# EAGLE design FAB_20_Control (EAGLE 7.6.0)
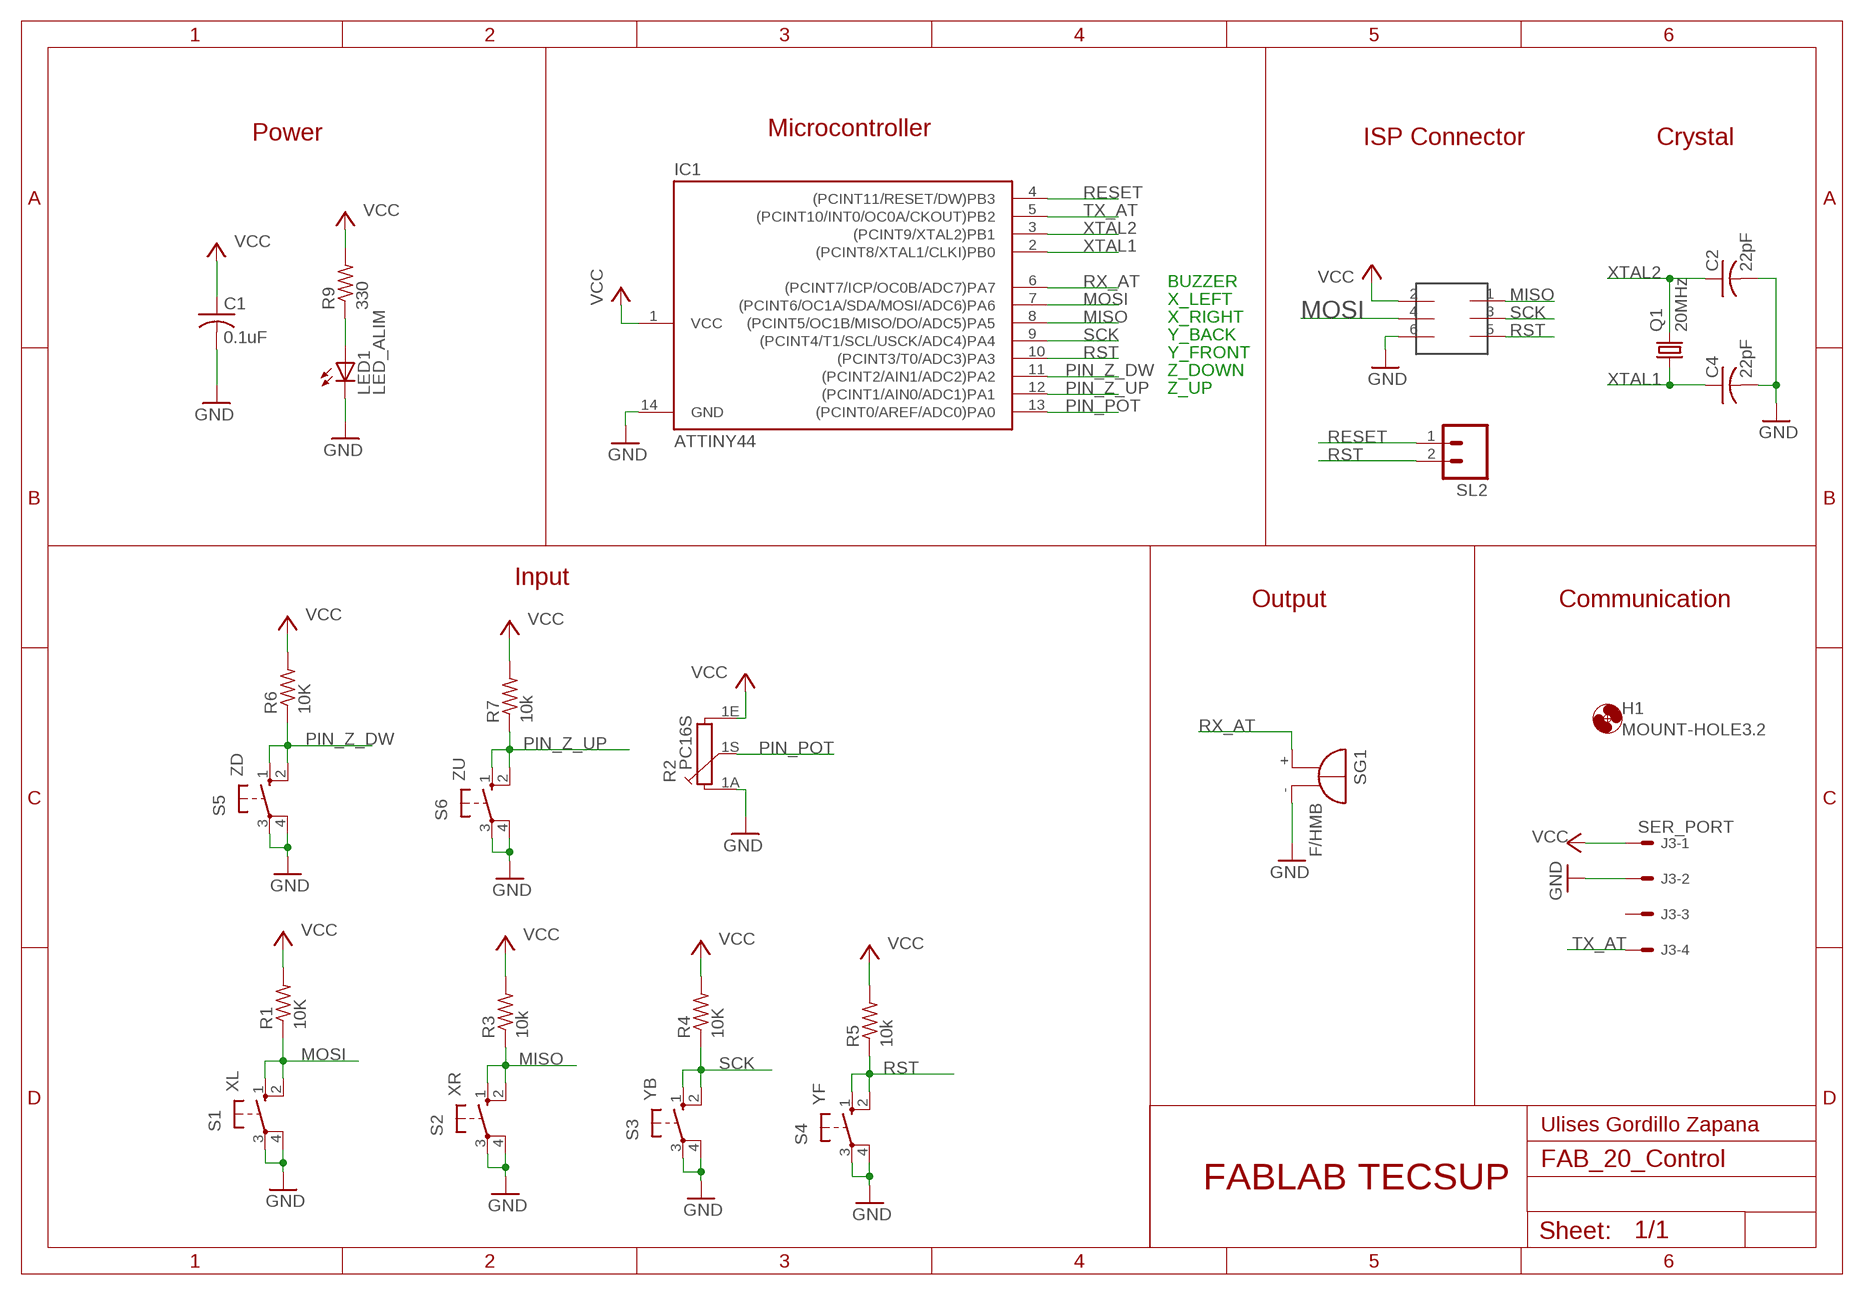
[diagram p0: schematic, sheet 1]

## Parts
C1  0.1uF  C-USC1206  [C1206]
C2  22pF  C-US025-030X050  [C025-030X050]
C4  22pF  C-US025-030X050  [C025-030X050]
H1  MOUNT-HOLE3.2  [3,2]
IC1  ATTINY44  ATTINY24/44/84-SSU  [SOIC14]
J3  SER_PORT  22-05-7048-04  [7395-04]
LED1  LED_ALIM  LED3MM  [LED3MM]
Q1  20MHz  CRYSTALHC49U-V  [HC49U-V]
R1  10K  R-US_R1206  [R1206]
R2  PC16S  [PC16S]
R3  10k  R-US_R1206  [R1206]
R4  10K  R-US_R1206  [R1206]
R5  10k  R-US_R1206  [R1206]
R6  10K  R-US_R1206  [R1206]
R7  10k  R-US_R1206  [R1206]
R9  330  R-US_R1206  [R1206]
S1  XL  10-XX  [B3F-10XX]
S2  XR  10-XX  [B3F-10XX]
S3  YB  10-XX  [B3F-10XX]
S4  YF  10-XX  [B3F-10XX]
S5  ZD  10-XX  [B3F-10XX]
S6  ZU  10-XX  [B3F-10XX]
SG1  F/HMB  [F/HMB]
SL2  M02  [02P]
U$1  2X3HEADER  [2X3_SMD]

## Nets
GND: C1.2 C2.2 C4.2 IC1.14(GND) J3.2 LED1.K(C) R2.1A S1.3(P) S1.4(P1) S2.3(P) S2.4(P1) S3.3(P) S3.4(P1) S4.3(P) S4.4(P1) S5.3(P) S5.4(P1) S6.3(P) S6.4(P1) SG1.- U$1.6
MISO: IC1.8((PCINT5/OC1B/MISO/DO/ADC5)PA5) R3.1 S2.1(S) S2.2(S1) U$1.1
MOSI: IC1.7((PCINT6/OC1A/SDA/MOSI/ADC6)PA6) R1.1 S1.1(S) S1.2(S1) U$1.4
N$8: LED1.A R9.1
PIN_POT: IC1.13((PCINT0/AREF/ADC0)PA0) R2.1S
PIN_Z_DW: IC1.11((PCINT2/AIN1/ADC2)PA2) R6.1 S5.1(S) S5.2(S1)
PIN_Z_UP: IC1.12((PCINT1/AIN0/ADC1)PA1) R7.1 S6.1(S) S6.2(S1)
RESET: IC1.4((PCINT11/RESET/DW)PB3) SL2.1
RST: IC1.10((PCINT3/T0/ADC3)PA3) R5.1 S4.1(S) S4.2(S1) SL2.2 U$1.5
RX_AT: IC1.6((PCINT7/ICP/OC0B/ADC7)PA7) SG1.+
SCK: IC1.9((PCINT4/T1/SCL/USCK/ADC4)PA4) R4.1 S3.1(S) S3.2(S1) U$1.3
TX_AT: IC1.5((PCINT10/INT0/OC0A/CKOUT)PB2) J3.4
VCC: C1.1 IC1.1(VCC) J3.1 R1.2 R2.1E R3.2 R4.2 R5.2 R6.2 R7.2 R9.2 U$1.2
XTAL1: C4.1 IC1.2((PCINT8/XTAL1/CLKI)PB0) Q1.1
XTAL2: C2.1 IC1.3((PCINT9/XTAL2)PB1) Q1.2
Unconnected: J3.3

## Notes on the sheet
- Power | Microcontroller
- ISP Connector | Crystal
- BUZZER
- X_LEFT
- X_RIGHT
- Y_BACK
- Y_FRONT
- Z_DOWN
- Z_UP
- Input
- Output | Communication
- Ulises Gordillo Zapana
- FABLAB TECSUP

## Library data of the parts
C1 = rcl-ez:C-US: CAPACITOR, American symbol
C2 C4 = rcl:C-US: CAPACITOR, American symbol
H1 = holes:MOUNT-HOLE: MOUNTING HOLE with drill center marker
IC1 = attiny24_44_84:ATTINY24/44/84
J3 = con-molex:22-?-04: CONNECTOR wire to board 2.54 mm (.1 inch) pitch header; OC_FARNELL: unknown; OC_NEWARK: unknown
LED1 = led:LED: LED
Q1 = crystal:CRYSTAL: CRYSTAL; OC_FARNELL: 1666969; OC_NEWARK: unknown
R1 R3-R7 R9 = rcl:R-US_: RESISTOR, American symbol
R2 = piher:PC16S: POTENTIOMETER single carbon potentiometer, 16 mm, S3ROH; OC_FARNELL: 4452940; OC_NEWARK: unknown
S1-S6 = switch-omron:10-XX: OMRON SWITCH; MPN: B3F-1000; OC_FARNELL: 176432; OC_NEWARK: 36M3542
SG1 = buzzer:F/HMB: BUZZER; OC_FARNELL: unknown; OC_NEWARK: unknown
SL2 = con-amp-quick:M02: AMP QUICK CONNECTOR; OC_FARNELL: unknown; OC_NEWARK: unknown
U$1 = mellis:2X3HEADER

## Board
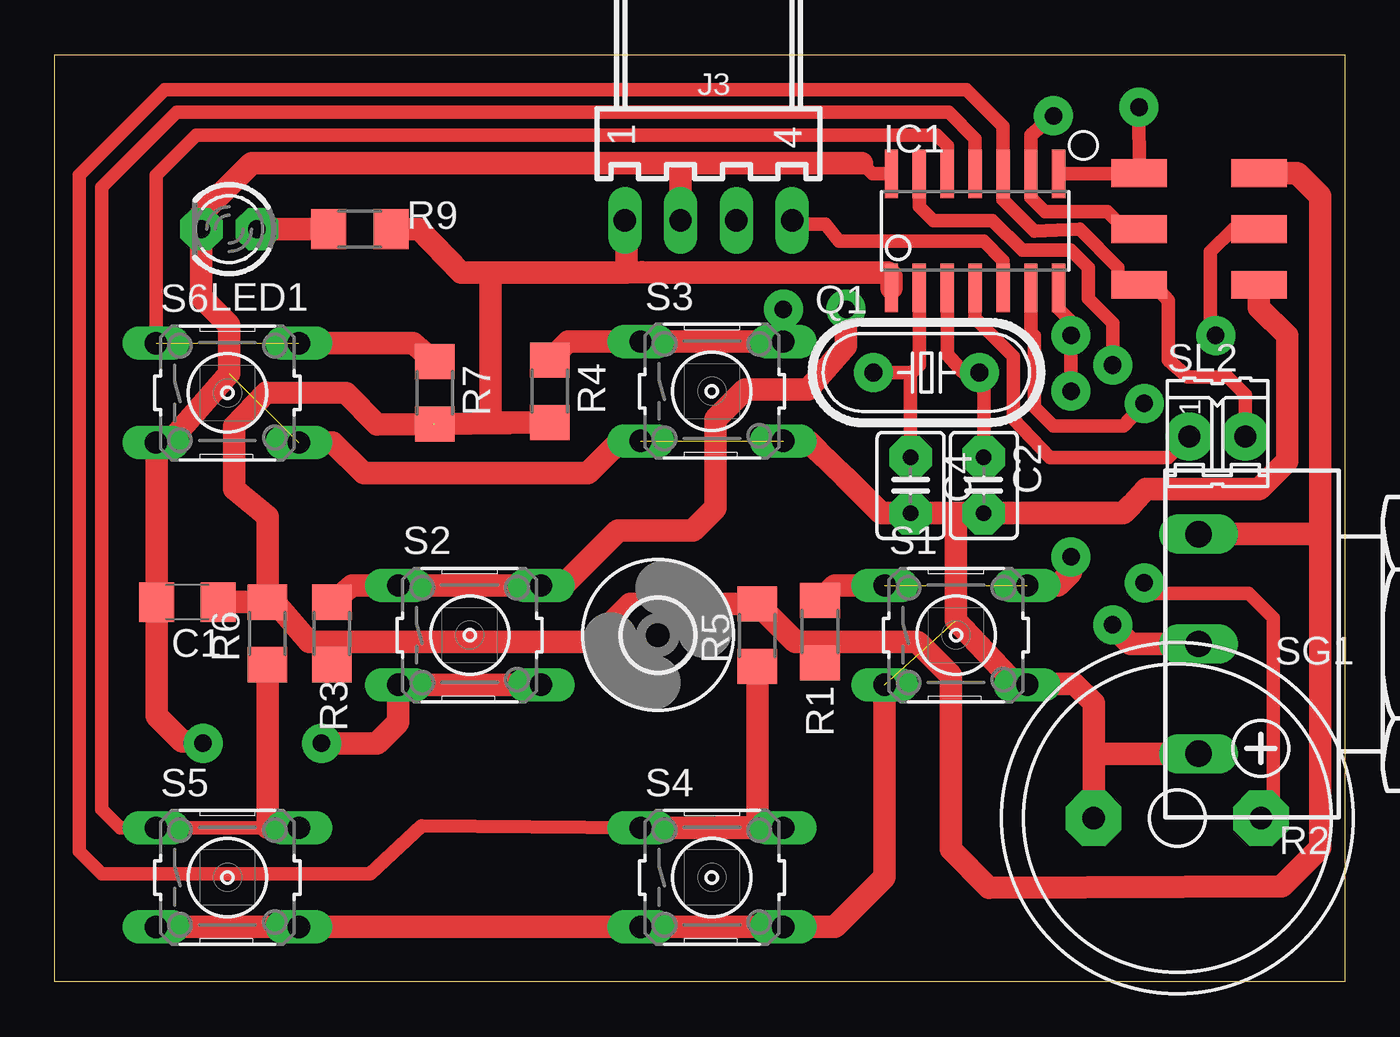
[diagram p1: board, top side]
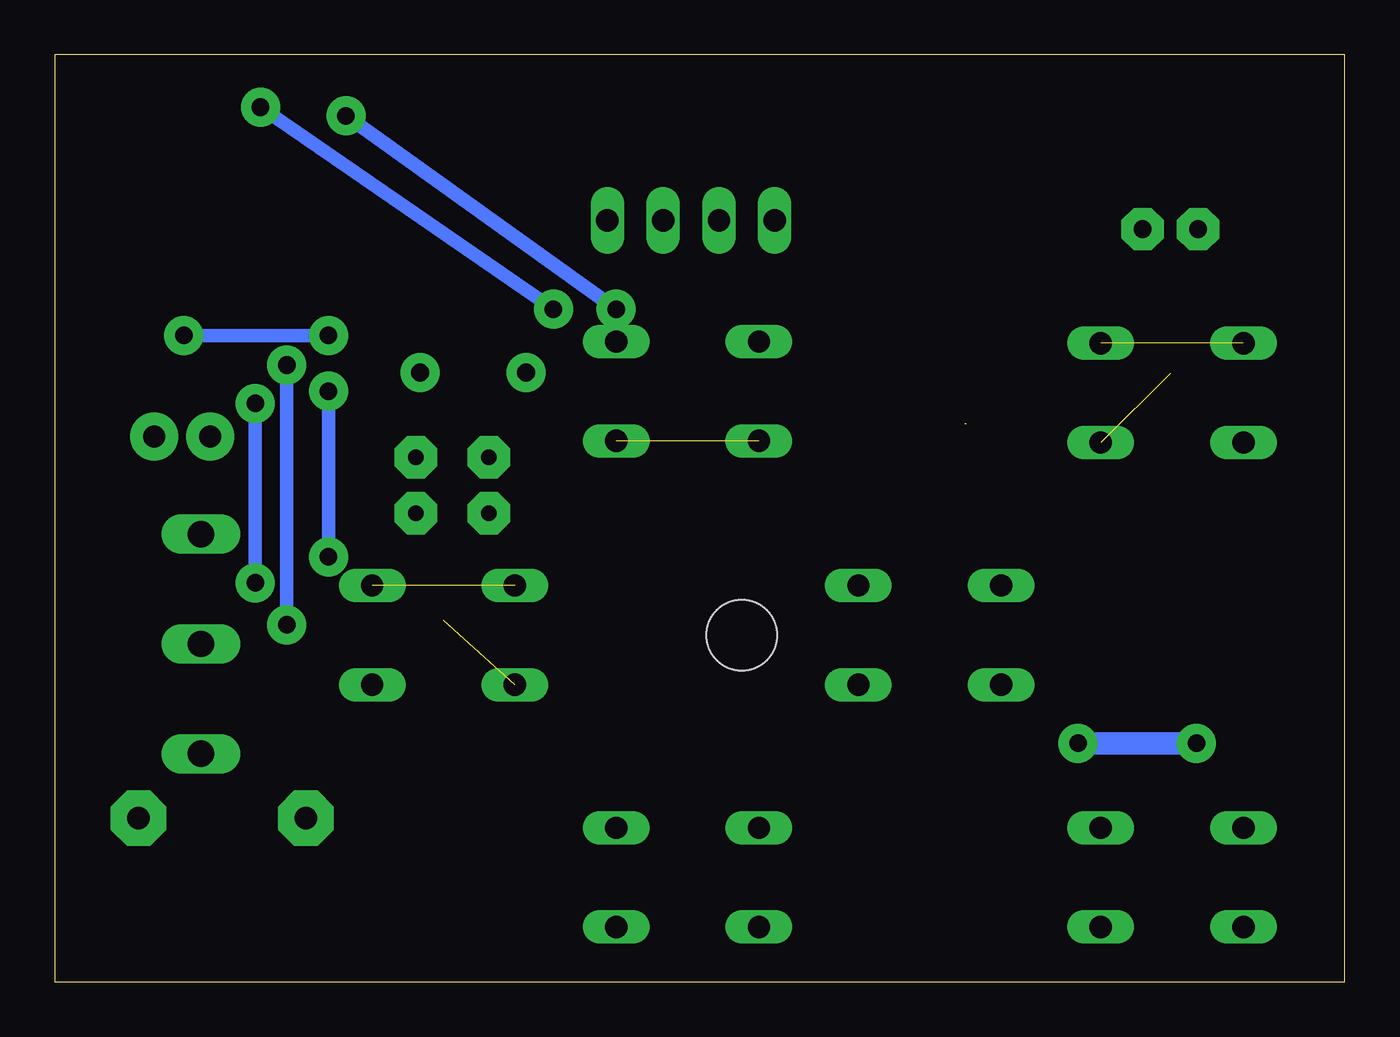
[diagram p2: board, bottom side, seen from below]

Size 58.74 x 42.23 mm. Coordinates in mm from the lower left corner, seen from the top.
Outline: 0,42.23 58.74,42.23 58.74,0 0,0 0,42.23
Copper layers (1*16): Top 0.035mm / dielectric 1.5mm / Bottom 0.035mm
Design rules "default *": minimum track width 12mil, minimum drill 24mil, track to track 17mil, track to pad 16mil, pad to pad 16mil, via to via 16mil, smd to smd 0mil, copper to edge 17mil, drill to drill 8mil, minimum pad ring 10mil, minimum via ring 8mil, stop-mask expansion 4mil, vias tented up to drill 0mil, thermal gap 10mil

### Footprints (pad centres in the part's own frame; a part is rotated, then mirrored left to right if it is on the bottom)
C1206 = smd 1.6 x 1.8: 1 -1.4,0; 2 1.4,0
C025-030X050 = drill 0.7 pad 1.93 octagon: 1 -1.27,0; 2 1.27,0
3,2 = hole 3.2: 0,0
SOIC14 = smd 0.61 x 2.21: 1 -3.81,-2.603; 2 -2.54,-2.603; 3 -1.27,-2.603; 4 0,-2.603; 5 1.27,-2.603; 6 2.54,-2.603; 7 3.81,-2.603; 8 3.81,2.603; 9 2.54,2.603; 10 1.27,2.603; 11 0,2.603; 12 -1.27,2.603; 13 -2.54,2.603; 14 -3.81,2.603
7395-04 = drill 1.016 long: 1 3.81,0; 2 1.27,0; 3 -1.27,0; 4 -3.81,0
LED3MM = drill 0.8 pad 1.93 octagon: A -1.27,0; K 1.27,0
HC49U-V = drill 0.813 pad 1.778: 1 -2.413,0; 2 2.413,0
R1206 = smd 1.6 x 1.803: 1 -1.422,0; 2 1.422,0
PC16S = drill 1.2 long: 1A -5,6.5; 1E 5,6.5; 1S 0,6.5
B3F-10XX = drill 1.016 long: 1 -3.251,2.261; 2 3.251,2.261; 3 -3.251,-2.261; 4 3.251,-2.261
F/HMB = drill 1.016 pad 2.54 octagon: + 3.81,0; - -3.81,0
02P = drill 1 pad 2.184: 1 -1.27,0; 2 1.27,0
2X3_SMD = smd 2.54 x 1.27: 1 -2.54,2.54; 2 2.92,2.54; 3 -2.54,0; 4 2.92,0; 5 -2.54,-2.54; 6 2.92,-2.54

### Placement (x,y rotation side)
C1  6.03,17.3 180 top
C2  42.31,22.62 270 top
C4  38.97,22.62 270 top
H1  27.46,15.8 0 top
IC1  41.91,34.21 0 top
J3  29.77,34.69 180 top
LED1  7.94,34.29 180 top
Q1  39.69,27.77 0 top
R1  34.85,15.95 270 top
R2  58.58,15.4 90 top
R3  12.62,15.88 270 top
R4  22.54,26.91 270 top
R5  31.99,15.8 90 top
R6  9.68,15.88 90 top
R7  17.3,26.83 270 top
R9  13.89,34.29 0 top
S1  41.04,15.8 0 top
S2  18.89,15.8 0 top
S3  29.92,26.91 0 top
S4  29.92,4.76 0 top
S5  7.86,4.76 0 top
S6  7.86,26.83 0 top
SG1  51.12,7.46 0 top
SL2  52.94,24.84 0 top
U$1  51.92,34.29 0 top

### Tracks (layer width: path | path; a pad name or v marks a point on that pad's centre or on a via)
GND  (via drill 0.8 pad 1.78)  (3 unrouted)
  Top 0.61: 44.33,13.57 S1.4 | IC1.14 37.24,36.81 36.75,37.31
  Top 1.016: R2.1A 47.31,10.4 | 47.31,10.4 47.31,12.7 46.43,13.57 44.33,13.57 | S5.3 S5.4 S4.3 S4.4 35.52,2.5 37.78,4.76 S1.3 | U$1.6 54.84,30.73 56.12,29.45 56.12,23.73 54.85,22.46 49.69,22.46 49.05,21.75 48.66,21.35 C2.2 41.04,21.35 | 28.5,37.29 8.95,37.29 6.67,35 LED1.K 6.67,31.19 7.94,29.92 7.94,27.7 5.16,24.53 4.65,24.53 S6.3 4.63,24.54 C1.2 4.63,12.12 5.79,10.95 6.67,10.95 v6.75,10.87 | J3.2 28.5,37.29 | S1.4 43.74,13.57 41.04,16.47 41.04,21.35 | v12.14,10.87 14.68,10.87 15.64,11.83 S2.3 S2.4 | S6.4 12.66,24.57 14.05,23.18 24.29,23.18 25.72,24.61 26.63,24.61 S3.3 | 36.75,37.31 28.51,37.31 28.5,37.29 | SG1.- 47.31,10.4 | 41.04,21.35 C4.2 37.62,21.35 35.96,23.02 34.77,24.17 34.29,24.65 S3.4
  Bottom 1.016: v12.14,10.87 v6.75,10.87
MISO  (via drill 0.8 pad 1.78)
  Top 0.61: IC1.8 49.04,36.81 U$1.1 v49.37,39.85
  Top 1.016: R3.1 13.54,18.06 S2.1 S2.2 23.14,18.06 25.64,20.56 29.05,20.56 30.08,21.59 30.08,25.64 31.43,26.99 34.29,26.99 36.04,28.97 v36.04,30.64
  Bottom 0.61: v36.04,30.64 v49.37,39.85
MOSI  (via drill 0.8 pad 1.78)  (1 unrouted)
  Top 0.61: U$1.4 53.66,34.29 52.63,33.26 52.63,29.69 v52.86,29.45 | v46.28,29.45 46.2,30.16 45.72,30.64 IC1.7 | v46.28,26.91 v46.28,29.45 | 46.28,29.69 v46.28,29.45
  Top 1.016: S1.1 35.52,18.06 R1.1 | S1.2 45.68,18.06 46.28,18.65 v46.28,19.37
  Bottom 0.61: v52.86,29.45 v46.28,29.45 | v46.28,19.37 v46.28,26.91
N$8
  Top 1.016: R9.1 LED1.A
PIN_POT  (via drill 0.8 pad 1.78)
  Top 0.61: IC1.13 39.37,35.32 40.01,34.69 42.7,34.69 44.05,33.34 46.28,33.34 47.07,32.54 47.07,31.11 48.18,30 v48.18,28.1
  Top 1.016: v48.18,16.27 48.18,16.19 48.97,15.4 R2.1S
  Bottom 0.61: v48.18,28.1 v48.18,16.27
PIN_Z_DW
  Top 0.61: IC1.11 41.91,38.42 40.72,39.61 5.56,39.61 2.14,36.2 2.14,7.86 2.98,7.02 S5.1 S5.2
  Top 1.016: R6.1 9.68,7.02 S5.2
PIN_Z_UP  (1 unrouted)
  Top 0.61: IC1.12 40.64,38.1 40.16,38.58 6.43,38.58 4.61,36.75 S6.1
  Top 1.016: S6.2 16.31,29.09 R7.1
RESET
  Top 0.61: IC1.4 41.91,30.24 43.66,28.5 43.66,25.64 45.32,23.89 50.72,23.89 SL2.1
RST
  Top 0.61: 49.05,31.75 48.42,31.75 48.42,32.54 46.67,34.29 44.61,34.21 43.18,35.64 IC1.10 43.18,38.97 41.51,40.64 5,40.64 1.11,36.75 1.11,5.95 2.14,4.92 14.37,4.92 16.71,7.1 S4.1 | 49.05,31.75 49.06,31.75 | 49.06,31.75 U$1.5 49.05,31.75 | SL2.2 54.21,26.75 53.42,27.54 51.59,27.54 50.72,28.34 50.72,31.04 50.01,31.83 49.21,31.83 49.13,31.75 49.06,31.75
  Top 1.016: S4.1 28.22,7.02 | 28.22,7.02 31.99,7.06 R5.1 | S4.2 28.22,7.02
RX_AT  (via drill 0.8 pad 1.78)
  Top 0.61: IC1.6 44.45,29.61 44.61,29.45 44.61,26.19 45.48,25.32 48.66,25.32 v49.61,26.35 | v49.61,18.18 50.01,17.7 54.37,17.7 55.48,16.59 55.48,8.02 SG1.+
  Bottom 0.61: v49.61,26.35 v49.61,18.18
SCK  (via drill 0.8 pad 1.78)
  Top 0.61: U$1.3 49.06,34.29 48.74,34.29 47.94,35.08 45.09,35.08 44.45,35.72 IC1.9 44.45,38.58 v45.48,39.45
  Top 1.016: v33.18,30.64 S3.2 S3.1 23.38,29.17 R4.1
  Bottom 0.61: v33.18,30.64 v45.48,39.45
TX_AT
  Top 0.61: IC1.5 43.18,32.86 42.31,33.73 35.72,33.73 35.08,34.53 33.73,34.53 J3.4
VCC  (1 unrouted)
  Top 1.016: R1.2 34.67,14.53 34.67,15.41 34.61,15.48 | 12.62,15.48 24.45,15.48 26.19,17.22 R5.2 33.73,15.48 34.61,15.48 | 12.62,15.48 11.58,15.48 10,17.3 R6.2 | 12.61,14.29 R3.2 12.62,15.48 | R6.2 9.68,21.19 8.18,22.46 8.18,25.32 9.61,26.84 13.26,26.83 14.68,25.4 17.22,25.41 R4.2 19.84,25.49 19.84,32.31 | IC1.1 38.1,32.15 37.94,32.31 27.86,32.31 26.73,32.32 26.04,32.31 | 26.04,32.31 26.04,34.61 J3.1 | U$1.2 56.59,36.83 57.63,35.8 57.63,20.24 | 57.63,20.24 57.63,6.11 55.88,4.37 42.55,4.29 40.8,6.03 40.8,13.97 39.29,15.48 34.61,15.48 | R2.1E | R2.1E 57.63,20.4 57.63,20.24 | R9.2 16.59,34.29 18.49,32.31 19.84,32.31 | 19.84,32.31 26.04,32.31 | C1.1 9.6,17.3 R6.2
XTAL1
  Top 0.61: Q1.1 39.04,27.77 | 39.04,27.77 39.37,28.1 IC1.2 | C4.1 38.97,27.75 39.04,27.77
XTAL2
  Top 0.61: IC1.3 40.64,28.57 41.35,27.78 41.93,27.78 | 41.93,27.78 Q1.2 | C2.1 42.31,27.3 42.07,27.78 41.93,27.78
